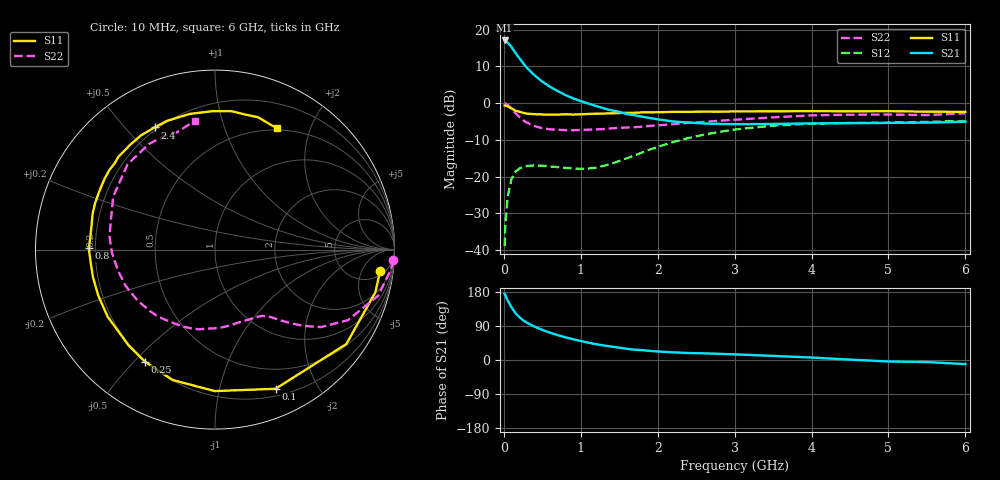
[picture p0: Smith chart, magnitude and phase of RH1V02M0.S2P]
! SIEMENS Small Signal Semiconductors
! BFR106
! Si NPN RF Bipolar Junction Transistor in SOT23
! VCE = 1 V  IC = 2 mA
! Common Emitter S-Parameters:  August  1996
# GHz  S  MA  R  50
!  f  S11  S21  S12  S22
! GHz  MAG  ANG  MAG  ANG  MAG  ANG  MAG  ANG
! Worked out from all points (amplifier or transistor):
!   36 points, 10 MHz to 6 GHz, reference 50 ohm
!   highest |S21| = 17.0 dB at 10 MHz (marker M1)
!   |S21| within 3 dB of that: start of sweep to 138 MHz
!   unconditionally stable (mu >= 1): 763.3 MHz to end of sweep
!   at 250 MHz: K = 0.34, MSG = 14.1 dB, |S12| = -17.4 dB
!   at 1.4 GHz: K = 1.37, MAG = 3.6 dB, |S12| = -16.5 dB
!   at 6 GHz: K = 1.03, MAG = -1.1 dB, |S12| = -4.9 dB
!   S11 on the Smith chart (normalised r, x): 10 MHz: 7, -12; 100 MHz: 0.27, -1.49; 250 MHz: 0.20, -0.54; 800 MHz: 0.17, +0.01; 2.4 GHz: 0.19, +0.61; 6 GHz: 0.48, +1.52
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0.01  0.9276 -7.4  7.106 174.6  0.0113 88.3  0.9955 -3.4
0.02  0.9246 -14.9  7.037 170.8  0.0222 83.5  0.9861 -6.6
0.05  0.9013 -35.7  6.627 156.8  0.0534 70.1  0.9443 -15.8
0.1  0.8456 -66.5  5.782 138.9  0.0927 54.3  0.8382 -28.0
0.15  0.7883 -90.1  4.815 123.8  0.1157 42.5  0.731 -36.2
0.2  0.7639 -108.0  4.105 113.6  0.1286 35.0  0.6491 -40.9
0.25  0.7362 -122.0  3.488 104.7  0.1355 29.2  0.5827 -44.5
0.3  0.7184 -132.3  3.01 98.5  0.1394 25.8  0.5424 -46.9
0.4  0.7053 -148.1  2.38 88.0  0.1421 20.8  0.4857 -50.6
0.5  0.6989 -158.7  1.954 79.4  0.1406 18.6  0.4544 -54.4
0.6  0.697 -167.6  1.664 72.1  0.1376 17.9  0.4396 -58.8
0.8  0.7034 179.4  1.286 59.9  0.1314 20.6  0.428 -68.3
1.1  0.7109 163.4  0.984 45.6  0.1285 32.3  0.4346 -84.5
1.6  0.7363 143.2  0.708 29.5  0.1779 52.0  0.4651 -112.8
2.2  0.7583 122.9  0.562 20.2  0.2944 52.1  0.5168 -146.8
2.4  0.7594 116.3  0.544 18.4  0.335 49.0  0.538 -158.2
3  0.769 100.6  0.516 14.9  0.4363 36.5  0.5928 172.7
3.5  0.7714 91.0  0.52 10.8  0.4931 25.9  0.6394 152.6
4.5  0.7711 77.0  0.533 1.0  0.5361 7.7  0.6935 122.2
5  0.7754 71.9  0.537 -3.9  0.5414 1.0  0.6979 111.0
5.5  0.7636 67.1  0.542 -5.4  0.5557 -2.2  0.6866 108.1
6  0.7595 63.1  0.557 -10.8  0.5699 -9.0  0.726 99.0
